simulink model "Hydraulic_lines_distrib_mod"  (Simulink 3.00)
settings: Solver=ode4  StartTime=0.0  StopTime=1.0  FixedStep=0.00005  MaxStep=0.01  RelTol=1e-3
StopFcn:
  | Final1
undefined symbols (not defined in the file or in its folder): Final, l, m3, s, to

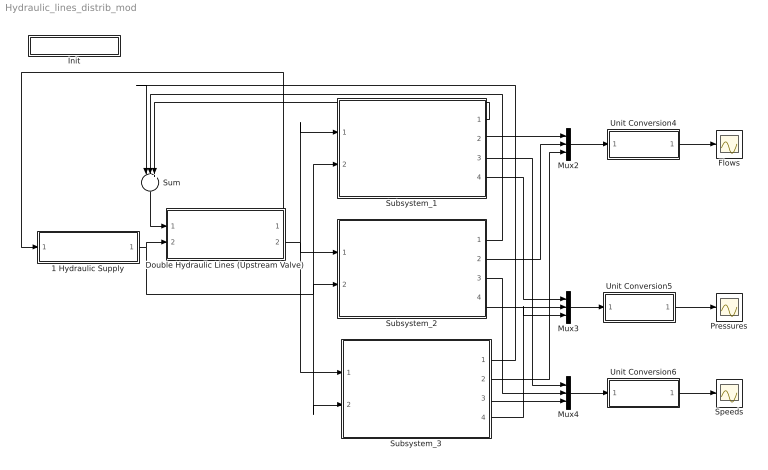
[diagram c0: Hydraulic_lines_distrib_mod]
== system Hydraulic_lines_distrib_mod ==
  1 Hydraulic Supply : Subsystem  mask(Variable Displacement Pump){Ps=20, Pr=0, rho_e=800, mu_e=15e-3, beta_e=900}
      mask prompts: Ps "System Supply Pressure [MPa]"; Pr "System Return Pressure [MPa]"; rho_e "Fluid density [kg/m3]"; mu_e "Fluid viscosity [kg/ms]"; beta_e "Bulk modulus [MPa]"
      mask help: Model of a variable displacement pump.
      mask init:
      | global rho
      | global mu
      | global beta
      | global beta1
      | rho=rho_e;
      | mu=mu_e;
      | beta=beta_e*1e6;
      | beta1=beta;
      | P_s = Ps*1.e6;
      | P_r = Pr*1.e6;
  Double Hydraulic Lines (Upstream Valve) : Subsystem  mask(Hydraulic Line){rl1=0, rl2=0, rq1=4.5e13, rq2=4.5e13, ll1=5, ll2=5, a1=7.85e-5, a2=7.85e-5}
      mask prompts: rl1 "Line 1 linear resistance coefficient [Pa s/m3]"; rl2 "Line 2 linear resistance coefficient [Pa s/m3]"; rq1 "Line 1 quadratic resistance coefficient [Pa s2/m6]"; rq2 "Line 2 quadratic resistance coefficient [Pa s2/m6]"; ll1 "Line 1 length [m]"; ll2 "Line 2  length [m]"; a1 "Line 1 section area [m2]"; a2 "Line 2 section area [m2]"
      mask init:
      | global rho
      | global beta
      | global beta1
      | L1 = rho*ll1/a1;
      | L2 = rho*ll2/a2;
      | C1=ll1*a1/beta1;
      | C2=ll2*a2/beta1;
  Flows : Scope
  Init : Subsystem  mask(Initialisation){Name_in=Final, Name_fin=Final, Ch=Unitialised Condition, Sav=off}
      mask prompts: Name_in "Initial state File Name"; Name_fin "Final state File Name"; Ch "Start from"; Sav "Save Current States to File"
      mask init:
      | global nome_f
      | global nome_i
      | 
      | 
      | if Ch==2
      |   set_param(gcs,'SaveFinalState','on')
      |   set_param(gcs,'FinalStateName','x_Final')
      |   set_param(gcs,'LoadInitialState','on')
      |   set_param(gcs,'InitialState','x_Final')
      | end
      | if Ch==3
      |   set_param(gcs,'LoadInitialState','off')
      |   set_param(gcs,'SaveFinalState','on')
      |   set_param(gcs,'FinalStateName','x_Final')
      | end
      | if Ch==1
      |   nome_i = Name_in;
      |     set_param(gcs,'InitialState','x_Initial')
      |     set_param(gcs,'LoadInitialState','on')
      |     set_param(gcs,'SaveFinalState','on')
      |     set_param(gcs,'FinalStateName','x_Final')
      |     run start_r
      | end
      | 
      | if Sav==1
      |   nome_f = Name_fin;
      |   set_param(gcs,'StopFcn','Initial1')
      | else
      |   set_param(gcs,'StopFcn','Final1')
      | end
  Mux2 : Mux  Inputs=3
  Mux3 : Mux  Inputs=3
  Mux4 : Mux  Inputs=3
  Pressures : Scope
  Speeds : Scope
  Subsystem_1 : Subsystem
  Subsystem_2 : Subsystem
  Subsystem_3 : Subsystem
  Sum : Sum  Orientation=down  Inputs=|+++  SaturateOnIntegerOverflow=on
  Unit Conversion4 : Subsystem  mask(Unit conversion){Ch=m3/s to l/min}
      mask prompts: Ch "Conversion type"
      mask init:
      | if Ch==1
      |   gain = 6e4;
      |  dsp = 'm3/s to l/min';
      | end
      | if Ch==2
      |   gain = 6.102e4;
      |   dsp = 'm3/s to cis';
      | end
      | if Ch==3
      |   gain = 15852;
      |   dsp = 'm3/s to gpm';
      | end
      | if Ch==4
      |   gain = 1e-6;
      |   dsp = 'Pa to MPa';
      | end
      | if Ch==5
      |   gain = 1.4503e-4;
      |   dsp = 'Pa to psi';
      | end
      | if Ch==6
      |   gain = 1000;
      |   dsp = 'm to mm';
      | end
      | if Ch==7
      |   gain = 39.37;
      |   dsp = 'm to in';
      | end
      | if Ch==8
      |   gain = 180/pi;
      |   dsp = 'rad to deg';
      | end
      | gain=1;
  Unit Conversion5 : Subsystem  mask(Unit conversion){Ch=Pa to MPa}
      mask prompts: Ch "Conversion type"
      mask init:
      | if Ch==1
      |   gain = 6e4;
      |  dsp = 'm3/s to l/min';
      | end
      | if Ch==2
      |   gain = 6.102e4;
      |   dsp = 'm3/s to cis';
      | end
      | if Ch==3
      |   gain = 15852;
      |   dsp = 'm3/s to gpm';
      | end
      | if Ch==4
      |   gain = 1e-6;
      |   dsp = 'Pa to MPa';
      | end
      | if Ch==5
      |   gain = 1.4503e-4;
      |   dsp = 'Pa to psi';
      | end
      | if Ch==6
      |   gain = 1000;
      |   dsp = 'm to mm';
      | end
      | if Ch==7
      |   gain = 39.37;
      |   dsp = 'm to in';
      | end
      | if Ch==8
      |   gain = 180/pi;
      |   dsp = 'rad to deg';
      | end
      | gain=1;
  Unit Conversion6 : Subsystem  mask(Unit conversion){Ch=rad to deg}
      mask prompts: Ch "Conversion type"
      mask init:
      | if Ch==1
      |   gain = 6e4;
      |  dsp = 'm3/s to l/min';
      | end
      | if Ch==2
      |   gain = 6.102e4;
      |   dsp = 'm3/s to cis';
      | end
      | if Ch==3
      |   gain = 15852;
      |   dsp = 'm3/s to gpm';
      | end
      | if Ch==4
      |   gain = 1e-6;
      |   dsp = 'Pa to MPa';
      | end
      | if Ch==5
      |   gain = 1.4503e-4;
      |   dsp = 'Pa to psi';
      | end
      | if Ch==6
      |   gain = 1000;
      |   dsp = 'm to mm';
      | end
      | if Ch==7
      |   gain = 39.37;
      |   dsp = 'm to in';
      | end
      | if Ch==8
      |   gain = 180/pi;
      |   dsp = 'rad to deg';
      | end
      | gain=1;
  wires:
  1 Hydraulic Supply/1(Pressures) -> Double Hydraulic Lines (Upstream Valve)/2(In_Pressures), Subsystem_2/2(Supply_Pressures), Subsystem_1/2(Supply_Pressures), Subsystem_3/2(Supply_Pressures)
  Double Hydraulic Lines (Upstream Valve)/2(Out_Pressures) -> Subsystem_2/1(In_Pressures), Subsystem_1/1(In_Pressures), Subsystem_3/1(In_Pressures)
  Unit Conversion5/1(Out1) -> Pressures/1
  Mux3/1 -> Unit Conversion5/1(Input)
  Subsystem_2/4(Out_Pressures) -> Mux3/2
  Subsystem_1/4(Out_Pressures) -> Mux3/1
  Subsystem_3/4(Out_Pressures) -> Mux3/3
  Subsystem_3/3(Speed) -> Mux4/3
  Unit Conversion6/1(Out1) -> Speeds/1
  Mux4/1 -> Unit Conversion6/1(Input)
  Subsystem_1/3(Speed) -> Mux4/1
  Subsystem_2/3(Speed) -> Mux4/2
  Subsystem_1/1(In_Flows) -> Sum/3
  Subsystem_1/2(Out_Flow) -> Mux2/1
  Subsystem_3/1(In_Flows) -> Sum/1
  Subsystem_3/2(Out_Flow) -> Mux2/3
  Double Hydraulic Lines (Upstream Valve)/1(In_Flows) -> 1 Hydraulic Supply/1(Out_Flow)
  Sum/1 -> Double Hydraulic Lines (Upstream Valve)/1(Out_Flows)
  Subsystem_2/2(Out_Flow) -> Mux2/2
  Subsystem_2/1(In_Flows) -> Sum/2
  Mux2/1 -> Unit Conversion4/1(Input)
  Unit Conversion4/1(Out1) -> Flows/1

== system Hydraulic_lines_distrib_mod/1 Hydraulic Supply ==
  Out_Flow : Inport  Port=1  PortWidth=-1  SampleTime=-1  DataType=auto
  Pressures : Outport  Port=1

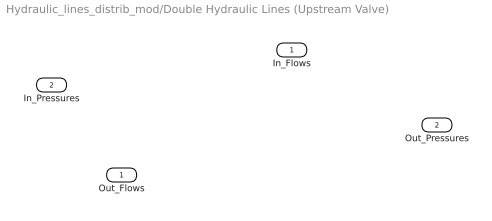
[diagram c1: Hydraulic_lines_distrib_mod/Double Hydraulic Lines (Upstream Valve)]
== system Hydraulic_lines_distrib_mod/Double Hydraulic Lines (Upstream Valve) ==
  Out_Flows : Inport  Port=1  PortWidth=-1  SampleTime=-1  DataType=auto
  In_Pressures : Inport  Port=2  PortWidth=-1  SampleTime=-1  DataType=auto
  In_Flows : Outport  Port=1
  Out_Pressures : Outport  Port=2
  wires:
  ? -> Out_Pressures/1
  Out_Flows/1 -> ?
  ? -> In_Flows/1
  In_Pressures/1 -> ?

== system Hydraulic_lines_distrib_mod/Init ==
  Subsystem : Subsystem

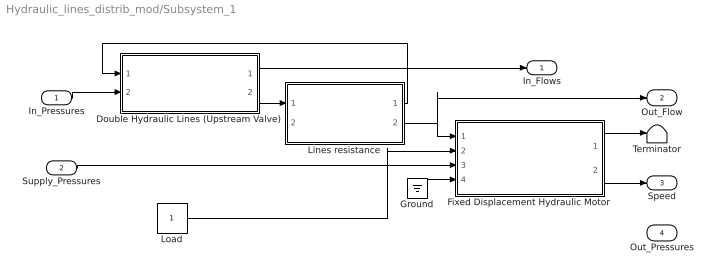
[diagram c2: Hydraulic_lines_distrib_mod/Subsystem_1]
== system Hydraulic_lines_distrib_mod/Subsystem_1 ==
  In_Pressures : Inport  Port=1  PortWidth=-1  SampleTime=-1  DataType=auto
  Supply_Pressures : Inport  Port=2  PortWidth=-1  SampleTime=-1  DataType=auto
  Double Hydraulic Lines (Upstream Valve) : Subsystem  mask(Hydraulic Line){rl1=0, rl2=0, rq1=4.5e13, rq2=4.5e13, ll1=5, ll2=5, a1=7.85e-5, a2=7.85e-5}
      mask prompts: rl1 "Line 1 linear resistance coefficient [Pa s/m3]"; rl2 "Line 2 linear resistance coefficient [Pa s/m3]"; rq1 "Line 1 quadratic resistance coefficient [Pa s2/m6]"; rq2 "Line 2 quadratic resistance coefficient [Pa s2/m6]"; ll1 "Line 1 length [m]"; ll2 "Line 2  length [m]"; a1 "Line 1 section area [m2]"; a2 "Line 2 section area [m2]"
      mask init:
      | global rho
      | global beta
      | global beta1
      | L1 = rho*ll1/a1;
      | L2 = rho*ll2/a2;
      | C1=ll1*a1/beta1;
      | C2=ll2*a2/beta1;
  Fixed Displacement Hydraulic Motor : Subsystem  mask(Hydraulic motor){Ds=3.33, Im=1.e-4, V0_out=1.67e-6, Cm=0, cfug=0, c_leak=0, Ploss=0, Cf=0, rkm=0, Ts=0, Td=0}
      mask prompts: Ds "Displacement [cc/rev]"; Im "Total Motor Inertia [kg*m2]"; V0_out "Hydraulic line volume [m3]"; Cm "Actuator Internal Damping [Nm/(rad/s)]"; cfug "Interport Leakage coeff. [(m3/s)/Pa]"; c_leak "Case Drain Leakage Coef. [(m3/s)/Pa]"; Ploss "Ploss (Help for definition)"; Cf "Cf (Help for definition)"; rkm "rkm (Help for definition)"; Ts "Static FrictionTorque [Nm]"; Td "Dynamic Friction Torque [Nm]"
      mask init:
      | global beta
      | D = Ds/1e6;
      | V0_in = V0_out;
  Ground : Ground
  Lines resistance : Subsystem  mask(Lines resistance){rq1=4.5e13, rl1=0, rq2=4.5e13, rl2=0}
      mask prompts: rq1 "Input line quadratic resistance [Pa/(m6/s2)]"; rl1 "Input line linear resistance [Pa/(m3/s)]"; rq2 "Output line quadratic resistance [Pa/(m6/s2)]"; rl2 "Output line linear resistance [Pa/(m3/s)]"
      mask init:
      | global rho
      | global mu
      | q_min=.01/60000;
  Load : Constant  Value=1
  Terminator : Terminator
  In_Flows : Outport  Port=1
  Out_Flow : Outport  Port=2
  Speed : Outport  Port=3
  Out_Pressures : Outport  Port=4
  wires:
  ? -> Out_Pressures/1, Lines resistance/2(Out_Pressures)
  Supply_Pressures/1 -> Fixed Displacement Hydraulic Motor/3(System_Pressures)
  In_Pressures/1 -> Double Hydraulic Lines (Upstream Valve)/2(In_Pressures)
  Double Hydraulic Lines (Upstream Valve)/2(Out_Pressures) -> Lines resistance/1(In_Pressures)
  Load/1 -> Fixed Displacement Hydraulic Motor/2(T_ext)
  Ground/1 -> Fixed Displacement Hydraulic Motor/4(Connection Torque)
  Fixed Displacement Hydraulic Motor/2(Speed) -> Speed/1
  Fixed Displacement Hydraulic Motor/1(Position) -> Terminator/1
  Double Hydraulic Lines (Upstream Valve)/1(In_Flows) -> In_Flows/1
  Lines resistance/2(Out_flows) -> Out_Flow/1, Fixed Displacement Hydraulic Motor/1(In_Flows)
  Lines resistance/1(In_Flows) -> Double Hydraulic Lines (Upstream Valve)/1(Out_Flows)

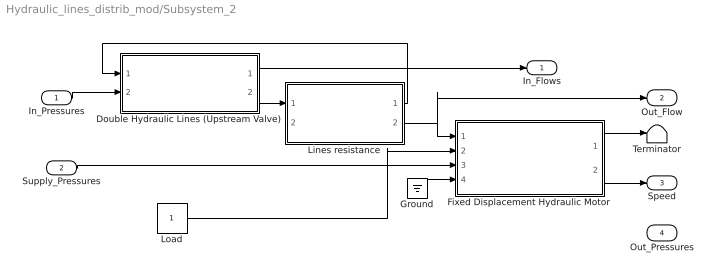
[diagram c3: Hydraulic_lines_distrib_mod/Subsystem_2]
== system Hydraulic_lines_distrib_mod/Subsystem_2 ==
  In_Pressures : Inport  Port=1  PortWidth=-1  SampleTime=-1  DataType=auto
  Supply_Pressures : Inport  Port=2  PortWidth=-1  SampleTime=-1  DataType=auto
  Double Hydraulic Lines (Upstream Valve) : Subsystem  mask(Hydraulic Line){rl1=0, rl2=0, rq1=4.5e13, rq2=4.5e13, ll1=5, ll2=5, a1=7.85e-5, a2=7.85e-5}
      mask prompts: rl1 "Line 1 linear resistance coefficient [Pa s/m3]"; rl2 "Line 2 linear resistance coefficient [Pa s/m3]"; rq1 "Line 1 quadratic resistance coefficient [Pa s2/m6]"; rq2 "Line 2 quadratic resistance coefficient [Pa s2/m6]"; ll1 "Line 1 length [m]"; ll2 "Line 2  length [m]"; a1 "Line 1 section area [m2]"; a2 "Line 2 section area [m2]"
      mask init:
      | global rho
      | global beta
      | global beta1
      | L1 = rho*ll1/a1;
      | L2 = rho*ll2/a2;
      | C1=ll1*a1/beta1;
      | C2=ll2*a2/beta1;
  Fixed Displacement Hydraulic Motor : Subsystem  mask(Hydraulic motor){Ds=3.33, Im=1.e-4, V0_out=1.67e-6, Cm=0, cfug=0, c_leak=0, Ploss=0, Cf=0, rkm=0, Ts=0, Td=0}
      mask prompts: Ds "Displacement [cc/rev]"; Im "Total Motor Inertia [kg*m2]"; V0_out "Hydraulic line volume [m3]"; Cm "Actuator Internal Damping [Nm/(rad/s)]"; cfug "Interport Leakage coeff. [(m3/s)/Pa]"; c_leak "Case Drain Leakage Coef. [(m3/s)/Pa]"; Ploss "Ploss (Help for definition)"; Cf "Cf (Help for definition)"; rkm "rkm (Help for definition)"; Ts "Static FrictionTorque [Nm]"; Td "Dynamic Friction Torque [Nm]"
      mask init:
      | global beta
      | D = Ds/1e6;
      | V0_in = V0_out;
  Ground : Ground
  Lines resistance : Subsystem  mask(Lines resistance){rq1=4.5e13, rl1=0, rq2=4.5e13, rl2=0}
      mask prompts: rq1 "Input line quadratic resistance [Pa/(m6/s2)]"; rl1 "Input line linear resistance [Pa/(m3/s)]"; rq2 "Output line quadratic resistance [Pa/(m6/s2)]"; rl2 "Output line linear resistance [Pa/(m3/s)]"
      mask init:
      | global rho
      | global mu
      | q_min=.01/60000;
  Load : Constant  Value=1
  Terminator : Terminator
  In_Flows : Outport  Port=1
  Out_Flow : Outport  Port=2
  Speed : Outport  Port=3
  Out_Pressures : Outport  Port=4
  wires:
  Lines resistance/1(In_Flows) -> Double Hydraulic Lines (Upstream Valve)/1(Out_Flows)
  Lines resistance/2(Out_flows) -> Fixed Displacement Hydraulic Motor/1(In_Flows), Out_Flow/1
  Double Hydraulic Lines (Upstream Valve)/1(In_Flows) -> In_Flows/1
  Fixed Displacement Hydraulic Motor/1(Position) -> Terminator/1
  Fixed Displacement Hydraulic Motor/2(Speed) -> Speed/1
  Ground/1 -> Fixed Displacement Hydraulic Motor/4(Connection Torque)
  Load/1 -> Fixed Displacement Hydraulic Motor/2(T_ext)
  Double Hydraulic Lines (Upstream Valve)/2(Out_Pressures) -> Lines resistance/1(In_Pressures)
  In_Pressures/1 -> Double Hydraulic Lines (Upstream Valve)/2(In_Pressures)
  Supply_Pressures/1 -> Fixed Displacement Hydraulic Motor/3(System_Pressures)
  ? -> Lines resistance/2(Out_Pressures), Out_Pressures/1

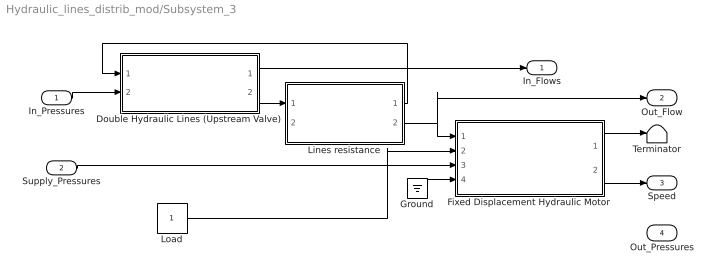
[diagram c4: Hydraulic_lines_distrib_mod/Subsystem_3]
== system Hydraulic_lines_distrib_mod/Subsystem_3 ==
  In_Pressures : Inport  Port=1  PortWidth=-1  SampleTime=-1  DataType=auto
  Supply_Pressures : Inport  Port=2  PortWidth=-1  SampleTime=-1  DataType=auto
  Double Hydraulic Lines (Upstream Valve) : Subsystem  mask(Hydraulic Line){rl1=0, rl2=0, rq1=4.5e13, rq2=4.5e13, ll1=5, ll2=5, a1=7.85e-5, a2=7.85e-5}
      mask prompts: rl1 "Line 1 linear resistance coefficient [Pa s/m3]"; rl2 "Line 2 linear resistance coefficient [Pa s/m3]"; rq1 "Line 1 quadratic resistance coefficient [Pa s2/m6]"; rq2 "Line 2 quadratic resistance coefficient [Pa s2/m6]"; ll1 "Line 1 length [m]"; ll2 "Line 2  length [m]"; a1 "Line 1 section area [m2]"; a2 "Line 2 section area [m2]"
      mask init:
      | global rho
      | global beta
      | global beta1
      | L1 = rho*ll1/a1;
      | L2 = rho*ll2/a2;
      | C1=ll1*a1/beta1;
      | C2=ll2*a2/beta1;
  Fixed Displacement Hydraulic Motor : Subsystem  mask(Hydraulic motor){Ds=3.33, Im=1.e-4, V0_out=1.67e-6, Cm=0, cfug=0, c_leak=0, Ploss=0, Cf=0, rkm=0, Ts=0, Td=0}
      mask prompts: Ds "Displacement [cc/rev]"; Im "Total Motor Inertia [kg*m2]"; V0_out "Hydraulic line volume [m3]"; Cm "Actuator Internal Damping [Nm/(rad/s)]"; cfug "Interport Leakage coeff. [(m3/s)/Pa]"; c_leak "Case Drain Leakage Coef. [(m3/s)/Pa]"; Ploss "Ploss (Help for definition)"; Cf "Cf (Help for definition)"; rkm "rkm (Help for definition)"; Ts "Static FrictionTorque [Nm]"; Td "Dynamic Friction Torque [Nm]"
      mask init:
      | global beta
      | D = Ds/1e6;
      | V0_in = V0_out;
  Ground : Ground
  Lines resistance : Subsystem  mask(Lines resistance){rq1=4.5e13, rl1=0, rq2=4.5e13, rl2=0}
      mask prompts: rq1 "Input line quadratic resistance [Pa/(m6/s2)]"; rl1 "Input line linear resistance [Pa/(m3/s)]"; rq2 "Output line quadratic resistance [Pa/(m6/s2)]"; rl2 "Output line linear resistance [Pa/(m3/s)]"
      mask init:
      | global rho
      | global mu
      | q_min=.01/60000;
  Load : Constant  Value=1
  Terminator : Terminator
  In_Flows : Outport  Port=1
  Out_Flow : Outport  Port=2
  Speed : Outport  Port=3
  Out_Pressures : Outport  Port=4
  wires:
  ? -> Out_Pressures/1, Lines resistance/2(Out_Pressures)
  Supply_Pressures/1 -> Fixed Displacement Hydraulic Motor/3(System_Pressures)
  In_Pressures/1 -> Double Hydraulic Lines (Upstream Valve)/2(In_Pressures)
  Double Hydraulic Lines (Upstream Valve)/2(Out_Pressures) -> Lines resistance/1(In_Pressures)
  Load/1 -> Fixed Displacement Hydraulic Motor/2(T_ext)
  Ground/1 -> Fixed Displacement Hydraulic Motor/4(Connection Torque)
  Fixed Displacement Hydraulic Motor/2(Speed) -> Speed/1
  Fixed Displacement Hydraulic Motor/1(Position) -> Terminator/1
  Double Hydraulic Lines (Upstream Valve)/1(In_Flows) -> In_Flows/1
  Lines resistance/2(Out_flows) -> Out_Flow/1, Fixed Displacement Hydraulic Motor/1(In_Flows)
  Lines resistance/1(In_Flows) -> Double Hydraulic Lines (Upstream Valve)/1(Out_Flows)

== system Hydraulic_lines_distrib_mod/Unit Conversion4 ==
  Input : Inport  Port=1  PortWidth=-1  SampleTime=-1  DataType=auto
  Gain : Gain  Gain=gain  SaturateOnIntegerOverflow=on
  Out1 : Outport  Port=1
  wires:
  Gain/1 -> Out1/1
  Input/1 -> Gain/1

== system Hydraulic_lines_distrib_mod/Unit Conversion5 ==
  Input : Inport  Port=1  PortWidth=-1  SampleTime=-1  DataType=auto
  Gain : Gain  Gain=gain  SaturateOnIntegerOverflow=on
  Out1 : Outport  Port=1
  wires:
  Input/1 -> Gain/1
  Gain/1 -> Out1/1

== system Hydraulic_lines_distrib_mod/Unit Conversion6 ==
  Input : Inport  Port=1  PortWidth=-1  SampleTime=-1  DataType=auto
  Gain : Gain  Gain=gain  SaturateOnIntegerOverflow=on
  Out1 : Outport  Port=1
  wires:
  Gain/1 -> Out1/1
  Input/1 -> Gain/1

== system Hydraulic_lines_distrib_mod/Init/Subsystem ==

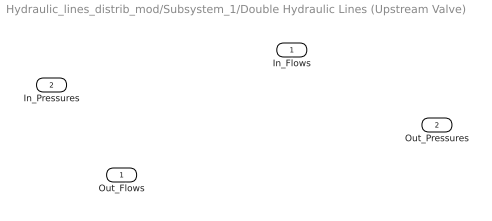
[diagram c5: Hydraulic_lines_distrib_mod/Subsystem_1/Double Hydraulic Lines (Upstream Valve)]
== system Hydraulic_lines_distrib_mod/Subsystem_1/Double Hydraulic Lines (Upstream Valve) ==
  Out_Flows : Inport  Port=1  PortWidth=-1  SampleTime=-1  DataType=auto
  In_Pressures : Inport  Port=2  PortWidth=-1  SampleTime=-1  DataType=auto
  In_Flows : Outport  Port=1
  Out_Pressures : Outport  Port=2
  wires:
  ? -> Out_Pressures/1
  Out_Flows/1 -> ?
  ? -> In_Flows/1
  In_Pressures/1 -> ?

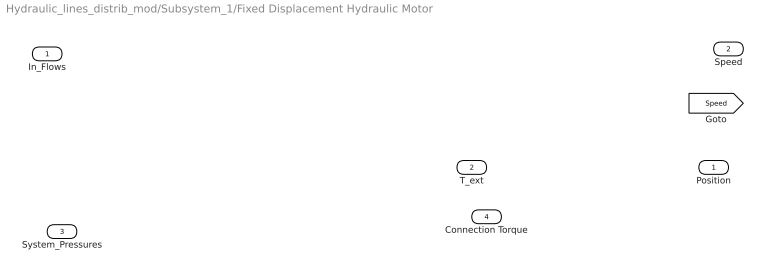
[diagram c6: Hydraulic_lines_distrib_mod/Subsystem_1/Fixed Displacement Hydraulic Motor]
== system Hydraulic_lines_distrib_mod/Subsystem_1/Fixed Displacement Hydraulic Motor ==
  In_Flows : Inport  Port=1  PortWidth=-1  SampleTime=-1  DataType=auto
  T_ext : Inport  Port=2  PortWidth=-1  SampleTime=-1  DataType=auto
  System_Pressures : Inport  Port=3  PortWidth=-1  SampleTime=-1  DataType=auto
  Connection Torque : Inport  Port=4  PortWidth=-1  SampleTime=-1  DataType=auto
  Position : Outport  Port=1
  Speed : Outport  Port=2
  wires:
  System_Pressures/1 -> ?
  In_Flows/1 -> ?
  ? -> Position/1
  Connection Torque/1 -> ?
  T_ext/1 -> ?
  ? -> [Speed], Speed/1

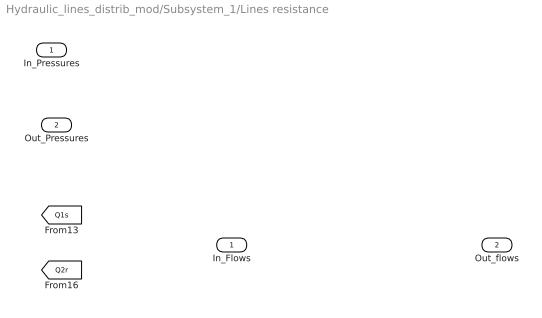
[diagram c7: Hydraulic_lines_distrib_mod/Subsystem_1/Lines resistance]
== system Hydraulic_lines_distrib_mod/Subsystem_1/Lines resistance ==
  In_Pressures : Inport  Port=1  PortWidth=-1  SampleTime=-1  DataType=auto
  Out_Pressures : Inport  Port=2  PortWidth=-1  SampleTime=-1  DataType=auto
  In_Flows : Outport  Port=1  InitialOutput=0
  Out_flows : Outport  Port=2  InitialOutput=0
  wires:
  In_Pressures/1 -> ?
  Out_Pressures/1 -> ?
  [Q1s] -> ?
  [Q2r] -> ?
  ? -> In_Flows/1
  ? -> Out_flows/1

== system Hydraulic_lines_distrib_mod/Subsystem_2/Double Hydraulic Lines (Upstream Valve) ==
  Out_Flows : Inport  Port=1  PortWidth=-1  SampleTime=-1  DataType=auto
  In_Pressures : Inport  Port=2  PortWidth=-1  SampleTime=-1  DataType=auto
  In_Flows : Outport  Port=1
  Out_Pressures : Outport  Port=2
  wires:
  In_Pressures/1 -> ?
  ? -> In_Flows/1
  Out_Flows/1 -> ?
  ? -> Out_Pressures/1

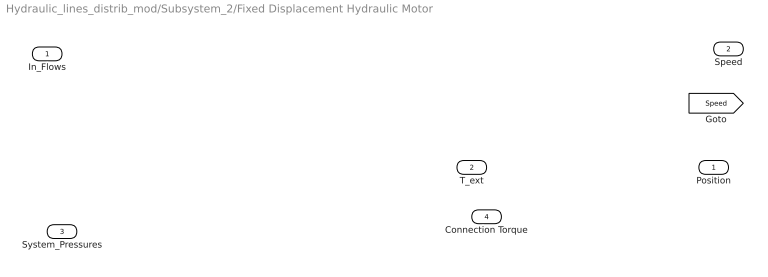
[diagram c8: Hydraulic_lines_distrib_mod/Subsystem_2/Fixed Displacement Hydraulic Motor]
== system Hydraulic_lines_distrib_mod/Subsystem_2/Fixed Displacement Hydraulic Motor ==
  In_Flows : Inport  Port=1  PortWidth=-1  SampleTime=-1  DataType=auto
  T_ext : Inport  Port=2  PortWidth=-1  SampleTime=-1  DataType=auto
  System_Pressures : Inport  Port=3  PortWidth=-1  SampleTime=-1  DataType=auto
  Connection Torque : Inport  Port=4  PortWidth=-1  SampleTime=-1  DataType=auto
  Position : Outport  Port=1
  Speed : Outport  Port=2
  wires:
  ? -> Speed/1, [Speed]
  T_ext/1 -> ?
  Connection Torque/1 -> ?
  ? -> Position/1
  In_Flows/1 -> ?
  System_Pressures/1 -> ?

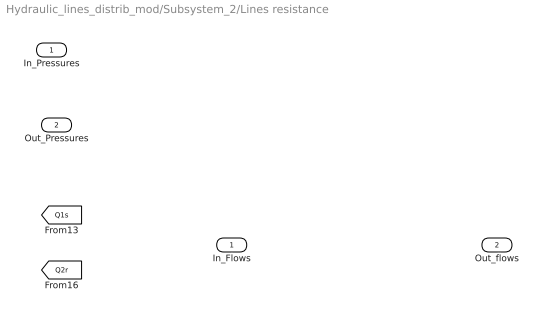
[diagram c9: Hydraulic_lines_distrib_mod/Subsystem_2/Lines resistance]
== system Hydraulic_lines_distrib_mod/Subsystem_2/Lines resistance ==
  In_Pressures : Inport  Port=1  PortWidth=-1  SampleTime=-1  DataType=auto
  Out_Pressures : Inport  Port=2  PortWidth=-1  SampleTime=-1  DataType=auto
  In_Flows : Outport  Port=1  InitialOutput=0
  Out_flows : Outport  Port=2  InitialOutput=0
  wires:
  ? -> Out_flows/1
  ? -> In_Flows/1
  [Q2r] -> ?
  [Q1s] -> ?
  Out_Pressures/1 -> ?
  In_Pressures/1 -> ?

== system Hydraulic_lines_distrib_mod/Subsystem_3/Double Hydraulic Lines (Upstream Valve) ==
  Out_Flows : Inport  Port=1  PortWidth=-1  SampleTime=-1  DataType=auto
  In_Pressures : Inport  Port=2  PortWidth=-1  SampleTime=-1  DataType=auto
  In_Flows : Outport  Port=1
  Out_Pressures : Outport  Port=2
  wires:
  ? -> Out_Pressures/1
  Out_Flows/1 -> ?
  ? -> In_Flows/1
  In_Pressures/1 -> ?

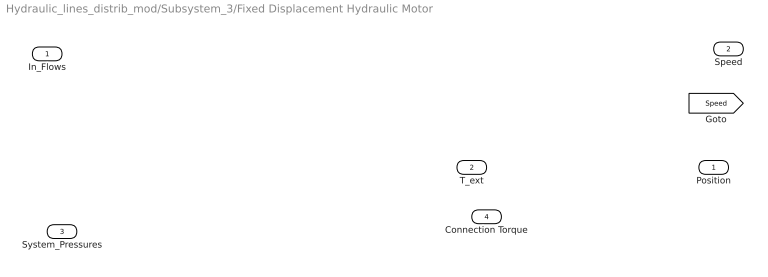
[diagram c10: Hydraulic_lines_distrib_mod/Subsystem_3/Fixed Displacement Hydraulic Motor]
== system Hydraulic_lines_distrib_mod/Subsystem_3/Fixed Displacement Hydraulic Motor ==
  In_Flows : Inport  Port=1  PortWidth=-1  SampleTime=-1  DataType=auto
  T_ext : Inport  Port=2  PortWidth=-1  SampleTime=-1  DataType=auto
  System_Pressures : Inport  Port=3  PortWidth=-1  SampleTime=-1  DataType=auto
  Connection Torque : Inport  Port=4  PortWidth=-1  SampleTime=-1  DataType=auto
  Position : Outport  Port=1
  Speed : Outport  Port=2
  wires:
  System_Pressures/1 -> ?
  In_Flows/1 -> ?
  ? -> Position/1
  Connection Torque/1 -> ?
  T_ext/1 -> ?
  ? -> [Speed], Speed/1

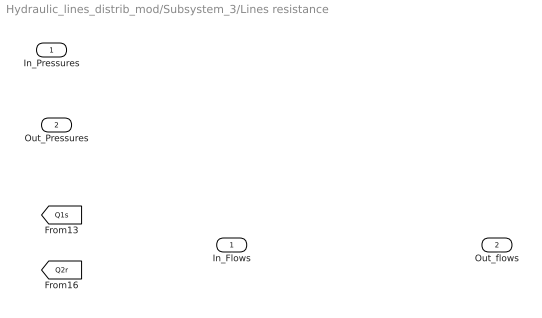
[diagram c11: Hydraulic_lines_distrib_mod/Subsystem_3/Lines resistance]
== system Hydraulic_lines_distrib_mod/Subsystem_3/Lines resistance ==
  In_Pressures : Inport  Port=1  PortWidth=-1  SampleTime=-1  DataType=auto
  Out_Pressures : Inport  Port=2  PortWidth=-1  SampleTime=-1  DataType=auto
  In_Flows : Outport  Port=1  InitialOutput=0
  Out_flows : Outport  Port=2  InitialOutput=0
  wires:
  In_Pressures/1 -> ?
  Out_Pressures/1 -> ?
  [Q1s] -> ?
  [Q2r] -> ?
  ? -> In_Flows/1
  ? -> Out_flows/1
